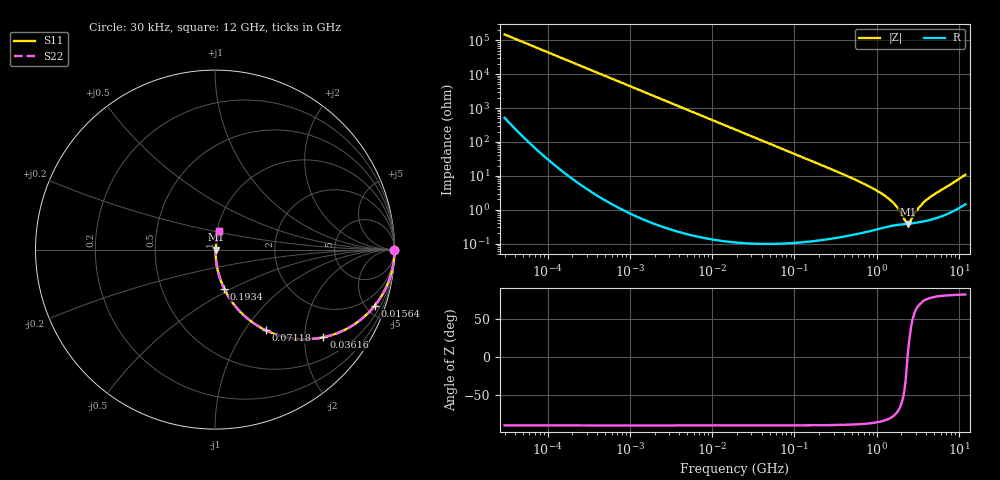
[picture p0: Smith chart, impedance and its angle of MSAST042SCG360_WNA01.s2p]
! MSAST042SCG360_WNA01  S-PARAMETER MODEL  ( General Type )
! Model Generated by TAIYO YUDEN Corporation (http://www.ty-top.com)
! Version 1.0
! TAIYO YUDEN Control No. 150820
! Copyright(c) 2015 TAIYO YUDEN CO.,LTD. All Rights Reserved.
! Product Description (link to TY-COMPAS)
! https://ds.yuden.co.jp/TYCOMPAS/or/detail?pn=MSAST042SCG360JWNA01&u=M
! Products Name : Multilayer Ceramic Capacitors
! Characteristics :
!  Capacitance : 36 pF , Rated Voltage : 25V , TCC : CG / C0G
!  Case Size : 0.4 x 0.2 / 0.016 x 0.008 [mm/inch] , Thickness : 0.2 / 0.008 [mm/inch]
!  (Conditions: Temperature = 25 degC , DC Bias Current/Voltage = 0A / 0V)
! External Node Assignments :
!  1  o---| |---o  2
! GND o---------o GND
! Frequency Range : 0.03MHz  -  12000MHz  [ 401 STEP ]
# MHz S RI R 50
! Freq[MHz].  S11 Real  S11 Imag  S21 Real  S21 Imag  S12 Real  S12 Imag  S22 Real  S22 Imag
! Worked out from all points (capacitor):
!   401 points, 30 kHz to 12 GHz, reference 50 ohm
!   read as one part in series: C = 35.7 pF near 32 kHz
!   lowest |Z| = 382 mohm at 2.393 GHz (marker M1)
!   series resonance near 2.376 GHz, so ESL is about 130 pH
!   S11 on the Smith chart (normalised r, x): 30 kHz: open; 15.64 MHz: 1.00, -5.71; 36.16 MHz: 1.00, -2.47; 71.18 MHz: 1.00, -1.25; 193.4 MHz: 1.00, -0.46; 12 GHz: 1.03, +0.21
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0.03  1 -0.000672  2.78e-06 0.000672  2.78e-06 0.000672  1 -0.000672
0.260295  1 -0.00583  3.58e-05 0.00583  3.58e-05 0.00583  1 -0.00583
2.258455  0.9974 -0.0505  0.00256 0.0505  0.00256 0.0505  0.9974 -0.0505
6.338349  0.9802 -0.1392  0.0198 0.1392  0.0198 0.1392  0.9802 -0.1392
15.63581  0.8906 -0.312  0.1094 0.312  0.1094 0.312  0.8906 -0.312
18.97367  0.8468 -0.3599  0.1532 0.3599  0.1532 0.3599  0.8468 -0.3599
36.16215  0.6035 -0.4888  0.3965 0.4888  0.3965 0.4888  0.6035 -0.4888
49.92358  0.4441 -0.4963  0.5559 0.4963  0.5559 0.4963  0.4441 -0.4963
71.18072  0.2822 -0.4493  0.7178 0.4493  0.7178 0.4493  0.2822 -0.4493
104.8152  0.1536 -0.3593  0.8464 0.3593  0.8464 0.3593  0.1536 -0.3593
164.6252  0.0688 -0.251  0.9312 0.251  0.9312 0.251  0.0688 -0.251
193.4292  0.051 -0.2173  0.949 0.2173  0.949 0.2173  0.051 -0.2173
725.66  0.00524 -0.0554  0.9948 0.0554  0.9948 0.0554  0.00524 -0.0554
1068.55  0.00383 -0.0332  0.9962 0.0332  0.9962 0.0332  0.00383 -0.0332
1428.372  0.00362 -0.02  0.9964 0.02  0.9964 0.02  0.00362 -0.02
1733.294  0.00365 -0.0122  0.9964 0.0122  0.9964 0.0122  0.00365 -0.0122
2243.435  0.00375 -0.00239  0.9963 0.00239  0.9963 0.00239  0.00375 -0.00239
2392.896  0.0038 0.000274  0.9962 -0.000274  0.9962 -0.000274  0.0038 0.000274
2552.314  0.00388 0.00228  0.9961 -0.00228  0.9961 -0.00228  0.00388 0.00228
3198.675  0.00429 0.00991  0.9957 -0.00991  0.9957 -0.00991  0.00429 0.00991
4008.724  0.00501 0.0185  0.995 -0.0185  0.995 -0.0185  0.00501 0.0185
12000  0.025 0.1026  0.975 -0.1026  0.975 -0.1026  0.025 0.1026
